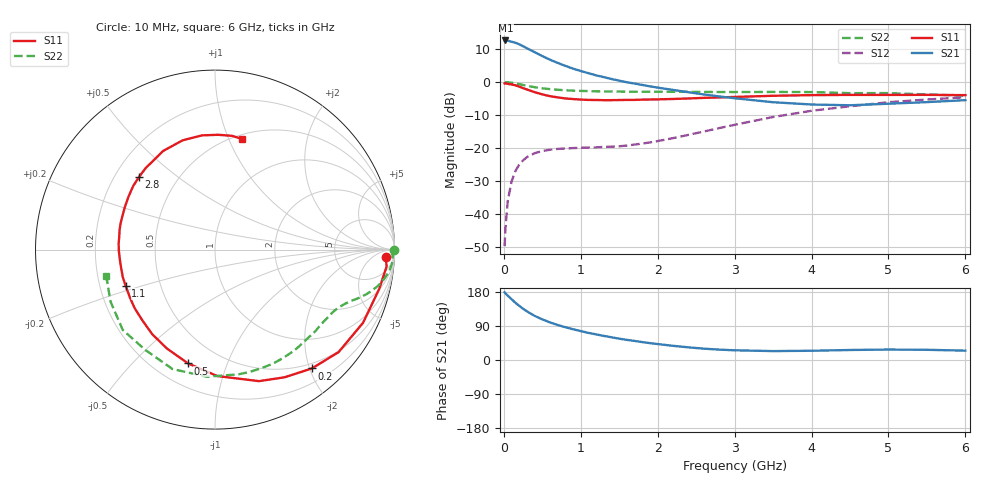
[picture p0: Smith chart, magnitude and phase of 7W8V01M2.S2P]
! Infineon Technologies  Discrete & RF Semiconductors
! BFS17W
! Si NPN RF Bipolar Junction Transistor in SOT323
! VCE = 8 V  IC = 1.2 mA
! Common Emitter S-Parameters:  August  1999
# GHz  S  MA  R  50
!  f  S11  S21  S12  S22
! GHz  MAG  ANG  MAG  ANG  MAG  ANG  MAG  ANG
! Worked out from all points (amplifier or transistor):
!   36 points, 10 MHz to 6 GHz, reference 50 ohm
!   highest |S21| = 12.6 dB at 20 MHz (marker M1)
!   |S21| within 3 dB of that: start of sweep to 354.4 MHz
!   unconditionally stable (mu >= 1): 1.014 GHz to 3.104 GHz; 4.1 GHz to end of sweep
!   at 250 MHz: K = 0.27, MSG = 17.3 dB, |S12| = -23.7 dB
!   at 1.4 GHz: K = 1.25, MAG = 7.2 dB, |S12| = -19.5 dB
!   at 6 GHz: K = 1.08, MAG = -2.2 dB, |S12| = -4.6 dB
!   S11 on the Smith chart (normalised r, x): 10 MHz: 22, -20; 200 MHz: 0.42, -2.04; 500 MHz: 0.33, -0.74; 1.1 GHz: 0.31, -0.18; 2.8 GHz: 0.30, +0.37; 6 GHz: 0.54, +1.12
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0.01  0.9518 -2.6  4.259 178.7  0.0033 84.4  0.9999 -0.2
0.02  0.9608 -5.6  4.262 176.1  0.006 89.7  0.989 -1.4
0.05  0.9411 -13.4  4.234 169.9  0.0157 83.6  0.9925 -3.6
0.1  0.9202 -26.3  4.083 160.6  0.0313 75.8  0.9791 -7.0
0.15  0.8947 -39.7  3.935 151.1  0.045 67.7  0.9552 -10.0
0.2  0.8542 -50.8  3.724 142.8  0.0567 62.9  0.9309 -12.5
0.25  0.8103 -61.4  3.491 135.2  0.0653 57.2  0.9031 -14.7
0.3  0.7728 -71.5  3.249 128.4  0.0734 52.8  0.8797 -16.4
0.4  0.7045 -89.0  2.836 116.5  0.0839 46.6  0.837 -19.1
0.5  0.6517 -103.3  2.472 107.2  0.0909 42.0  0.8051 -21.0
0.6  0.6128 -115.9  2.179 99.1  0.0948 39.2  0.7826 -22.8
0.7  0.587 -126.5  1.95 92.4  0.0976 37.9  0.7653 -24.6
0.9  0.554 -143.9  1.598 81.1  0.1005 36.9  0.7423 -28.2
1.1  0.5371 -157.8  1.363 71.5  0.1026 38.7  0.7302 -32.1
1.6  0.538 176.4  0.993 53.0  0.1097 49.0  0.7152 -43.0
2.2  0.5555 154.7  0.761 37.4  0.1421 63.6  0.7132 -57.9
2.8  0.5859 136.2  0.607 27.4  0.2015 70.0  0.7083 -74.2
3.5  0.6209 117.7  0.496 23.5  0.2964 68.4  0.7098 -93.7
4  0.635 106.5  0.458 24.4  0.3683 63.0  0.7063 -109.6
4.5  0.6405 96.5  0.446 26.4  0.4306 56.3  0.6807 -124.8
5.5  0.6409 81.6  0.498 26.9  0.5453 42.4  0.6501 -153.6
6  0.6349 76.2  0.533 24.7  0.5889 35.7  0.6234 -166.4
